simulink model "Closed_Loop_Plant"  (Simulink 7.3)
settings: Solver=ode23s  StartTime=0.0  StopTime=30  FixedStep=0.04  RelTol=1e-3
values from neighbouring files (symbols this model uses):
  Ap = Au([3,4,7,9,10],[3,4,7,9,10])    [Split.m]
  Bp = Bu([3,4,7,9,10],                      [4,8, 10,12,13,15,16,17,18,23,25,27,31,32,33,34])    [Split.m]
  Cp = Cu([3,4,7,9,10,12,14, 16,18,19,21,22,23,24,29,31,33,37,38,39,40],         [3,4,7,9,10])    [Split.m]
  Dp = Du([3,4,7,9,10,12,14, 16,18,19,21,22,23,24,29,31,33,37,38,39,40],                      [4,8, 10,12,13,15,16,17,18,23,25,27,31,32,33,34])    [Split.m]
  r2d = 180/pi    (= 57.2957795131)    [run.m]    (also in Pl.m; pl.m; start.m)
undefined symbols (not defined in the file or in its folder): Ac, Bc, Cc, Dc

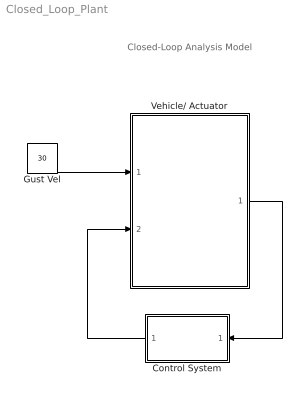
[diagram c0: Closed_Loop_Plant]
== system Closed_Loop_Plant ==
  note: Closed-Loop Analysis Model
  Control System : Subsystem
  Gust Vel : Constant  Value=30  OutDataType=sfix(16)  OutScaling=2^0
  Vehicle/ Actuator : Subsystem
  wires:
  Gust Vel/1 -> Vehicle/ Actuator/1(Vgust)
  Vehicle/ Actuator/1(control) -> Control System/1(control)
  Control System/1(TVC) -> Vehicle/ Actuator/2(TVC)

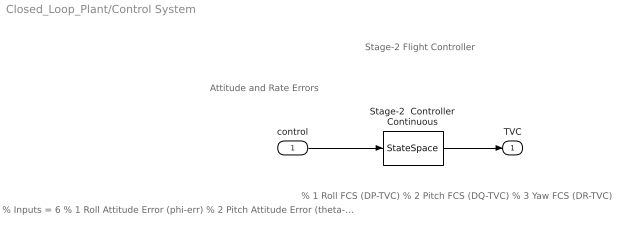
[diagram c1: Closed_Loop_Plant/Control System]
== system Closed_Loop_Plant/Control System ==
  note: Stage-2 Flight Controller
  note: Attitude and Rate Errors
  note: % Inputs = 6 % 1 Roll Attitude Error (phi-err) % 2 Pitch Attitude Error (theta-err) % 3 Yaw Attitude Error (psi-err) % 4 Roll Rate Error (p-err) % 5 Pitch Rate Error (q-err) % 6 Yaw Rate Error (r-err)
  note: % 1 Roll FCS (DP-TVC) % 2 Pitch FCS (DQ-TVC) % 3 Yaw FCS (DR-TVC)
  control : Inport  OutDataType=sfix(16)  OutScaling=2^0
  Stage-2  Controller Continuous : StateSpace  A=Ac  B=Bc  C=Cc  D=Dc
  TVC : Outport  OutDataType=sfix(16)  OutScaling=2^0
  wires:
  control/1 -> Stage-2  Controller Continuous/1
  Stage-2  Controller Continuous/1 -> TVC/1

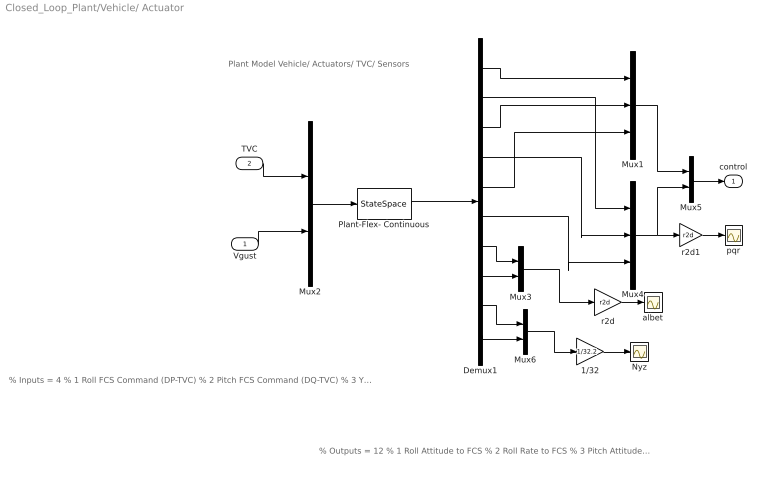
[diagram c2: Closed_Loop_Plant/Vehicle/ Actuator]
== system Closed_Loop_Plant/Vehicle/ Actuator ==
  note: Plant Model Vehicle/ Actuators/ TVC/ Sensors
  note: % Inputs = 4 % 1 Roll FCS Command (DP-TVC) % 2 Pitch FCS Command (DQ-TVC) % 3 Yaw FCS Command (DR-TVC) % 4 Wind-Gust Velocity (ft/sec)
  note: % Outputs = 12 % 1 Roll Attitude to FCS % 2 Roll Rate to FCS % 3 Pitch Attitude to FCS % 4 Pitch Rate to FCS % 5 Yaw Attitude to FCS % 6 Yaw Rate to FCS % 7 Angle of Attack, alpha (rad) % 8 Angle of Sideslip, beta (rad) % 9 Normal Accelerometer, Nz (ft/sec^2) % 10 Lateral Accelerometer, Ny (ft/sec^2)
  Vgust : Inport  OutDataType=sfix(16)  OutScaling=2^0
  TVC : Inport  Port=2  OutDataType=sfix(16)  OutScaling=2^0
  1/32 : Gain  Gain=1/32.2  ParameterDataType=sfix(16)  ParameterScaling=2^0  OutDataType=sfix(16)  OutScaling=2^0
  Demux1 : Demux  Outputs=10
  Mux1 : Mux  Inputs=3
  Mux2 : Mux  Inputs=[3, 1]
  Mux3 : Mux  Inputs=2
  Mux4 : Mux  Inputs=3
  Mux5 : Mux  Inputs=2
  Mux6 : Mux  Inputs=2
  Nyz : Scope
  Plant-Flex- Continuous : StateSpace  A=Ap  B=Bp  C=Cp  D=Dp
  albet : Scope
  pqr : Scope
  r2d : Gain  Gain=r2d  ParameterDataType=sfix(16)  ParameterScaling=2^0  OutDataType=sfix(16)  OutScaling=2^0
  r2d1 : Gain  Gain=r2d  ParameterDataType=sfix(16)  ParameterScaling=2^0  OutDataType=sfix(16)  OutScaling=2^0
  control : Outport  OutDataType=sfix(16)  OutScaling=2^0
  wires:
  Mux6/1 -> 1/32/1
  Mux2/1 -> Plant-Flex- Continuous/1
  Plant-Flex- Continuous/1 -> Demux1/1
  Demux1/9 -> Mux6/1
  Demux1/10 -> Mux6/2
  Demux1/8 -> Mux3/2
  Demux1/7 -> Mux3/1
  Demux1/6 -> Mux4/3
  Demux1/4 -> Mux4/2
  Demux1/2 -> Mux4/1
  Demux1/3 -> Mux1/2
  Demux1/5 -> Mux1/3
  Demux1/1 -> Mux1/1
  Mux1/1 -> Mux5/1
  Mux4/1 -> Mux5/2, r2d1/1
  Mux5/1 -> control/1
  TVC/1 -> Mux2/1
  Vgust/1 -> Mux2/2
  Mux3/1 -> r2d/1
  r2d/1 -> albet/1
  1/32/1 -> Nyz/1
  r2d1/1 -> pqr/1
